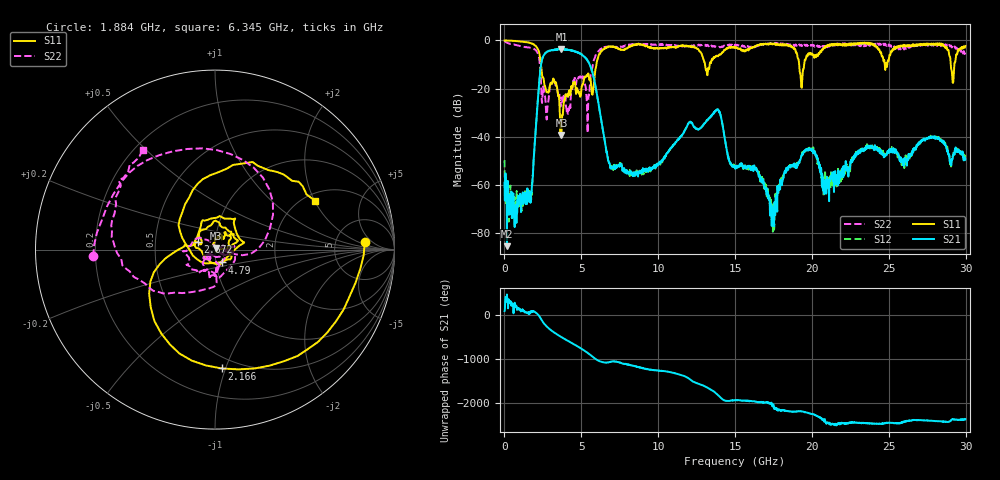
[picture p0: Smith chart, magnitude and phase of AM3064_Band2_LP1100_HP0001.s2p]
# Hz S DB R 50.0
!freq dBS11 angS11 dBS21 angS21 dBS12 angS12 dBS22 angS22
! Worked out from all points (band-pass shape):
!   1600 points, 10 MHz to 29.98 GHz, reference 50 ohm
!   highest |S21| = -3.64 dB at 3.703 GHz (marker M1); lowest = -85.3 dB at 159.9 MHz (marker M2)
!   |S21| within 3 dB of the highest: 2.519 GHz to 5.183 GHz (2.664 GHz wide, 69.2 % of centre)
!   lowest |S11| = -39.3 dB at 3.703 GHz (marker M3), VSWR 1.02, Z = 50.7 + j0.847 ohm
!   |S11| at or under -10 dB: 2.373 GHz to 5.982 GHz (3.609 GHz wide, 86.4 % of centre); 13.04 GHz to 13.35 GHz (304.8 MHz wide, 2.31 % of centre); 19.17 GHz to 19.49 GHz (324.4 MHz wide, 1.68 % of centre)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
!   |S22| runs from -38.4 to -0.3 dB; largest |S21 - S12| = 0.018
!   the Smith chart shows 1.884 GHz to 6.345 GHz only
!   S11 on the Smith chart (normalised r, x): 1.884 GHz: 10, +3; 2.166 GHz: 0.41, -0.97; 2.672 GHz: 0.82, +0.07; 4.79 GHz: 1.07, -0.15; 6.345 GHz: 2.28, +2.02
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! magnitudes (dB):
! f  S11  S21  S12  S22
! 10 MHz  -0.1  -59.2  -49.7  -0.3
! 159.9 MHz  -0.1  -85.3  -62.3  -0.9
! 1.603 GHz  -1.0  -64.7  -62.5  -3.0
! 1.884 GHz  -1.6  -50.9  -50.9  -3.4
! 2.166 GHz  -3.6  -25.2  -25.2  -5.4
! 2.672 GHz  -19.7  -5.2  -5.2  -25.4
! 3.703 GHz  -39.3  -3.6  -3.8  -24.0
! 4.79 GHz  -21.7  -5.0  -5.0  -15.9
! 5.015 GHz  -19.5  -5.8  -5.9  -16.4
! 5.427 GHz  -14.1  -8.7  -8.5  -31.2
! 6.345 GHz  -4.1  -35.2  -35.0  -3.3
! 7.001 GHz  -2.7  -52.9  -53.0  -2.7
! 10 GHz  -3.4  -51.7  -50.9  -1.8
! 13.82 GHz  -6.4  -28.7  -28.8  -2.6
! 15 GHz  -2.8  -53.2  -52.8  -1.9
! 16.39 GHz  -2.2  -53.5  -53.2  -2.4
! 17.46 GHz  -1.3  -69.8  -79.3  -1.3
! 19.33 GHz  -19.6  -47.4  -47.7  -2.2
! 19.99 GHz  -5.5  -45.4  -45.2  -1.9
! 20.97 GHz  -2.6  -56.5  -57.8  -2.2
! 25 GHz  -8.0  -46.3  -46.1  -1.7
! 29.98 GHz  -2.3  -49.2  -48.5  -4.8
